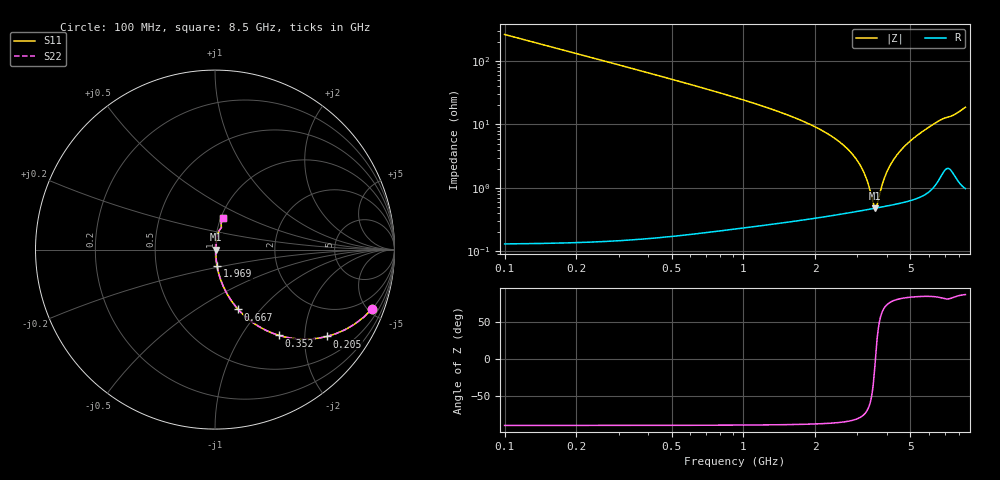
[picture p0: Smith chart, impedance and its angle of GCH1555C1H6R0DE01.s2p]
!Murata Part Number: GCH1555C1H6R0DE01
!These Parameters are Measured in Series Mode Connection
!Data Generated on Mar 13, 2026
!  o--ll--o
!Port1  Port2
!  o------o
!Operation Temp=25[degC], DC Bias Voltage=0[V]
!Freq. Start=100[MHz] Stop=9[GHz] 401[Steps]
# Hz S RI R 50
!Freq.(Hz) S11(Real) S11(Imag) S21(Real) S21(Imag) S12(Real) S12(Imag) S22(Real) S22(Imag)
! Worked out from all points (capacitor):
!   401 points, 100 MHz to 8.5 GHz, reference 50 ohm
!   read as one part in series: C = 6 pF near 142 MHz
!   lowest |Z| = 475 mohm at 3.565 GHz (marker M1)
!   series resonance near 3.571 GHz, so ESL is about 330 pH
!   S11 on the Smith chart (normalised r, x): 100 MHz: 1.00, -5.30; 205 MHz: 1.00, -2.58; 352 MHz: 1.00, -1.49; 667 MHz: 1.00, -0.77; 1.969 GHz: 1.01, -0.19; 8.5 GHz: 1.02, +0.37
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1e8  0.8753 -0.3302  0.1247 0.3302  0.1247 0.3302  0.8753 -0.3302
2.05e8  0.6243 -0.4838  0.3757 0.4838  0.3757 0.4838  0.6243 -0.4838
3.52e8  0.3578 -0.4783  0.6422 0.4783  0.6422 0.4783  0.3578 -0.4783
4.99e8  0.2141 -0.4086  0.7859 0.4086  0.7859 0.4086  0.2141 -0.4086
6.67e8  0.1294 -0.3332  0.8706 0.3332  0.8706 0.3332  0.1294 -0.3332
9.82e8  0.0605 -0.2338  0.9395 0.2338  0.9395 0.2338  0.0605 -0.2338
1.507e9  0.0232 -0.141  0.9768 0.141  0.9768 0.141  0.0232 -0.141
1.969e9  0.0119 -0.0926  0.9881 0.0926  0.9881 0.0926  0.0119 -0.0926
2.536e9  0.00647 -0.0517  0.9935 0.0517  0.9935 0.0517  0.00647 -0.0517
2.914e9  0.00506 -0.0305  0.9949 0.0305  0.9949 0.0305  0.00506 -0.0305
3.229e9  0.00464 -0.0151  0.9954 0.0151  0.9954 0.0151  0.00464 -0.0151
3.355e9  0.00462 -0.00936  0.9954 0.00936  0.9954 0.00936  0.00462 -0.00936
3.502e9  0.00467 -0.00292  0.9953 0.00292  0.9953 0.00292  0.00467 -0.00292
3.565e9  0.00472 -0.000234  0.9953 0.000234  0.9953 0.000234  0.00472 -0.000234
3.628e9  0.00478 0.00241  0.9952 -0.00241  0.9952 -0.00241  0.00478 0.00241
3.796e9  0.00502 0.00929  0.995 -0.00929  0.995 -0.00929  0.00502 0.00929
3.922e9  0.00525 0.0143  0.9947 -0.0143  0.9947 -0.0143  0.00525 0.0143
4.3e9  0.00624 0.0287  0.9938 -0.0287  0.9938 -0.0287  0.00624 0.0287
4.867e9  0.00846 0.0491  0.9915 -0.0491  0.9915 -0.0491  0.00846 0.0491
5.707e9  0.0138 0.0786  0.9862 -0.0786  0.9862 -0.0786  0.0138 0.0786
7.114e9  0.0349 0.121  0.9651 -0.121  0.9651 -0.121  0.0349 0.121
8.5e9  0.0425 0.1775  0.9575 -0.1775  0.9575 -0.1775  0.0425 0.1775
